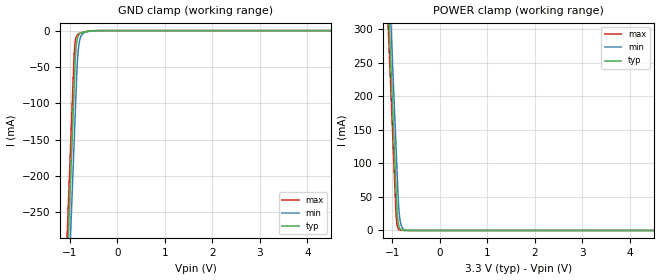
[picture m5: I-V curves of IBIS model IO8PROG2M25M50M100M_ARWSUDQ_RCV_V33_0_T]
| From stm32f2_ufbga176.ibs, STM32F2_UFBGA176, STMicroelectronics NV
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| *** New cell (Generated with 5.14beta1 (Sep 20 2010 13:23:23))
[Model]   IO8PROG2M25M50M100M_ARWSUDQ_RCV_V33_0_T
Model_type Input
Polarity   Non-Inverting
Enable   Active-Low
| CAP_THRESHOLD on pad IOV33 is "CMOS" :
| Rising=10.0% of vddio   Falling=90.0% of vddio
| C_comp min and max val. don't necessarily correlate with the min and max pvt
| but are the smallest and greatest pad capacitance found.
| var   typ   min   max
C_comp   2.45405pF  2.36060pF  2.57685pF
Vinl = 800.0mV | Dummy value overriden by next lines
Vinh = 2.00V | Dummy value overriden by next lines
[Model Spec]
| TIME_THRESHOLD on pin ZIV33 is "CORE" :
| Rising=40.0% of vddio   Falling=60.0% of vddio
Vinl 1.25450V 1.03850V 1.36250V
Vinh 1.66150V 1.36950V 1.82450V
| variable   typ   min   max
[Temperature Range] 25.0 125.0 -40.0
| variable   typ   min   max
[Voltage Range] 3.3V 2.7V 3.6V
| variable   typ   min   max
[POWER Clamp Reference] 3.3V 2.7V 3.6V
| variable   typ   min   max
[GND Clamp Reference] 0V 0V 0V
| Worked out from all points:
|   GND clamp passes 1 mA (typ) near -0.62 V on its own axis
|   POWER clamp passes 1 mA (typ) near -0.81 V on its own axis
[POWER Clamp]
-3.3V     4.11A      4.173A     4.072A
-1.09V    352.6mA    415.9mA    314.7mA
-1.05V    284.6mA    347.9mA    246.7mA
-1.01V    216.6mA    279.9mA    178.7mA
-920mV    63.6mA     126.9mA    25.98mA
-900mV    31.61mA    92.95mA    9.679mA
-890mV    21.44mA    75.95mA    5.93mA
-870mV    9.888mA    44.06mA    2.262mA
-840mV    3.126mA    18.4mA     586.7uA
-780mV    356.4uA    3.233mA    107.9uA
-660mV    37.87uA    120.8uA    47.09uA
6.6V      0A         0A         0A
[GND Clamp]
-3.3V     -4.149A    -4.224A    -4.103A
-1.06V    -340.8mA   -415.7mA   -294.7mA
-940mV    -136.8mA   -211.7mA   -90.7mA
-900mV    -68.75mA   -143.7mA   -26.69mA
-880mV    -36.92mA   -109.7mA   -13.58mA
-870mV    -26.73mA   -92.66mA   -10.38mA
-840mV    -11.43mA   -45.13mA   -6.003mA
-820mV    -7.322mA   -27.2mA    -4.821mA
-790mV    -4.504mA   -13.49mA   -3.791mA
-700mV    -1.961mA   -2.954mA   -1.882mA
-350mV    -6.427uA   -36.3uA    -1.194uA
6.6V      9.775nA    1.217uA    66.58pA
